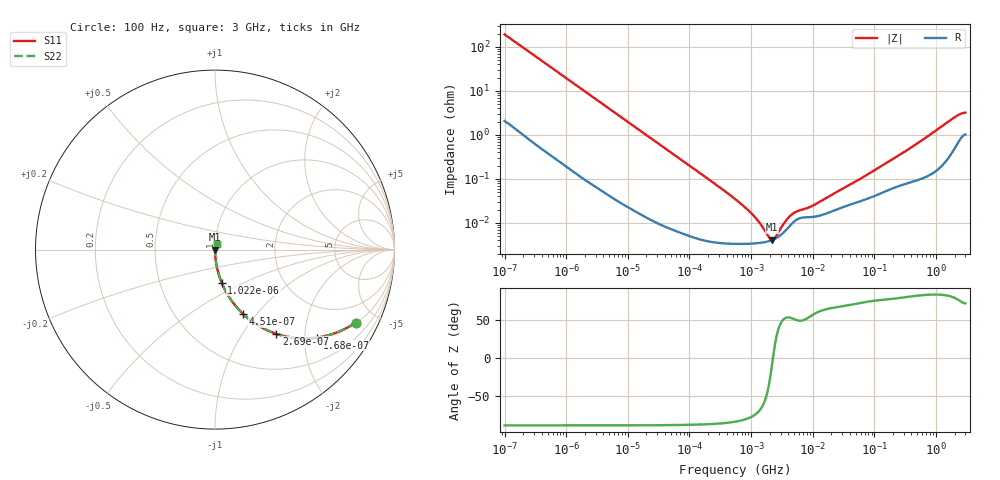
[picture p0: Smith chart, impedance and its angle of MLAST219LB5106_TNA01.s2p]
! MLAST219LB5106_TNA01  S-PARAMETER MODEL  ( Standard Model )
! Model Generated by TAIYO YUDEN Corporation (http://www.ty-top.com)
! Version 1.0
! TAIYO YUDEN Control No. 220601
! Copyright(c) 2014 TAIYO YUDEN CO.,LTD. All Rights Reserved.
! Product Description (link to TY-COMPAS)
! https://ds.yuden.co.jp/TYCOMPAS/or/detail?pn=MLAST219LB5106KTNA01&u=M
! Products Name : Multilayer Ceramic Capacitors
! Characteristics :
!  Capacitance : 10 [uF] , Rated Voltage : 25 [V] , TCC : X5R
!  Case Size : 2.0 x 1.25 / 0.079 x 0.049 [mm/inch] , Thickness : 0.85 / 0.033 [mm/inch]
!  (Conditions: Temperature = 25 [degC] , DC Bias Voltage = 0 [V])
! External Node Assignments :
!  1  o---| |---o  2
! GND o---------o GND
! Frequency Range : 100Hz  -  3GHz  [ 401 STEP ]
# MHZ S RI R 50
! Freq[MHz].  S11 Real  S11 Imag  S21 Real  S21 Imag  S12 Real  S12 Imag  S22 Real  S22 Imag
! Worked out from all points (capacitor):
!   401 points, 100 Hz to 3 GHz, reference 50 ohm
!   read as one part in series: C = 8.28 uF near 109 Hz
!   lowest |Z| = 4.12 mohm at 2.171 MHz (marker M1)
!   series resonance near 2.266 MHz, so ESL is about 600 pH
!   S11 on the Smith chart (normalised r, x): 100 Hz: 1.04, -3.84; 168 Hz: 1.02, -2.30; 269 Hz: 1.01, -1.44; 451 Hz: 1.01, -0.86; 1.022 kHz: 1.00, -0.38; 3 GHz: 1.02, +0.06
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0.0001  0.784 -0.4062  0.216 0.4062  0.216 0.4062  0.784 -0.4062
0.000168  0.5686 -0.49  0.4314 0.49  0.4314 0.49  0.5686 -0.49
0.000269  0.3419 -0.4694  0.6581 0.4694  0.6581 0.4694  0.3419 -0.4694
0.000451  0.1584 -0.3603  0.8416 0.3603  0.8416 0.3603  0.1584 -0.3603
0.000664  0.0811 -0.2681  0.9189 0.2681  0.9189 0.2681  0.0811 -0.2681
0.001022  0.0368 -0.1834  0.9632 0.1834  0.9632 0.1834  0.0368 -0.1834
0.001788  0.0128 -0.1078  0.9872 0.1078  0.9872 0.1078  0.0128 -0.1078
0.005476  0.00167 -0.0359  0.9983 0.0359  0.9983 0.0359  0.00167 -0.0359
0.031977  0.000133 -0.00622  0.9999 0.00622  0.9999 0.00622  0.000133 -0.00622
0.547723  3.34e-05 -0.000348  1 0.000348  1 0.000348  3.34e-05 -0.000348
0.87939  3.35e-05 -0.000196  1 0.000196  1 0.000196  3.35e-05 -0.000196
1.352413  3.49e-05 -9.72e-05  1 9.72e-05  1 9.72e-05  3.49e-05 -9.72e-05
1.53882  3.58e-05 -7.17e-05  1 7.17e-05  1 7.17e-05  3.58e-05 -7.17e-05
2.171352  4.05e-05 -7.8e-06  1 7.8e-06  1 7.8e-06  4.05e-05 -7.8e-06
3.339322  5.97e-05 7.18e-05  0.9999 -7.18e-05  0.9999 -7.18e-05  5.97e-05 7.18e-05
5.135543  0.000111 0.000133  0.9999 -0.000133  0.9999 -0.000133  0.000111 0.000133
9.794414  0.000136 0.000201  0.9999 -0.000201  0.9999 -0.000201  0.000136 0.000201
54.78865  0.000299 0.000895  0.9997 -0.000895  0.9997 -0.000895  0.000299 0.000895
175.1444  0.000573 0.00246  0.9994 -0.00246  0.9994 -0.00246  0.000573 0.00246
492.0662  0.000965 0.00625  0.999 -0.00625  0.999 -0.00625  0.000965 0.00625
2036.508  0.00569 0.0248  0.9943 -0.0248  0.9943 -0.0248  0.00569 0.0248
3000  0.011 0.0298  0.989 -0.0298  0.989 -0.0298  0.011 0.0298
